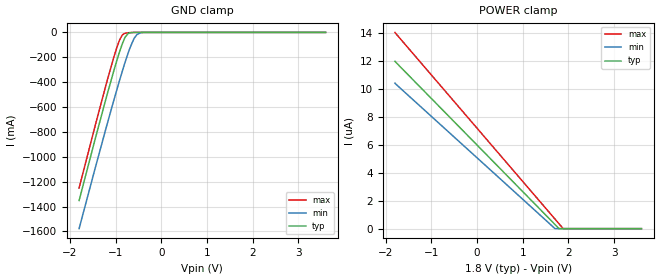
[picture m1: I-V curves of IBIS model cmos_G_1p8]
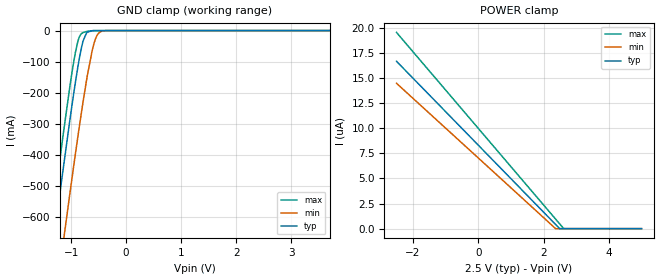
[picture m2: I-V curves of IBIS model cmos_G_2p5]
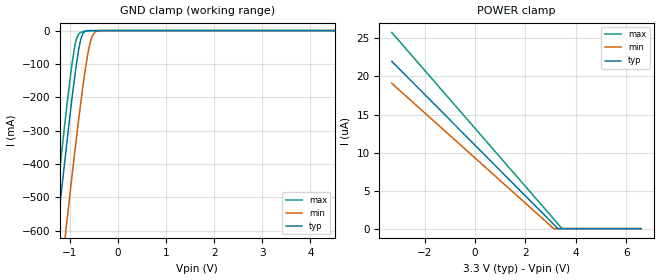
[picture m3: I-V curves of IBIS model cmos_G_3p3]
|Texas Instruments Incorporated
| 1.8V, 2.5V, 3.3V LVCMOS High-Performance Clock Buffer
| Marketing Part # : LMK1C1104
| Voltage Range : 1.71V-3.465V
| Package-type: TSSOP
| #pins/pkg drawing : 8-pin TSSOP
[IBIS Ver] 4.1
[File name] lmk1c1104.ibs
[File Rev] 1.0
[Date] 12/03/2019
[Source]
| Texas Instruments Incorporated.
| 12500 TI Blvd
| Dallas, TX -75243
[Notes] Revision History:
| Rev 1.0: 12/03/2019
| - Initial version of the model
| - Model generated from simulations in SPECTRE
| - C_comp although listed in numerical order of value are
| obtained from varying PVT conditions. For PVT conditions for
| each specific value refer the buffer description under
| respective [Model]. IBIS model user is responsible for using
| appropriate C_comp to simulate for Signal Integrity.
| - Warnings regarding combined Non-monotonicity of various models have been
| reviewed and considered minor and can be ignored.
| - Model names with a trailing _1p8 contain the model for
| 1.8V operation. Model names with a trailing _2p5 contain the model
| for 2.5V operation. Model names with a trailing _3p3 contain the model
| for 3.3V operation.
[Disclaimer]
| This model is designed as an aid for customers of Texas Instruments.
| TI and its licensors and suppliers make no warranties, either expressed
| or implied, with respect to this model, including the warranties of
| merchantability or fitness for a particular purpose. The model is
| provided solely on an "as is" basis. The entire risk as to its quality
| and performance is with the customer.
| This model is subject to change without notice. Texas Instruments
| Incorporated is not responsible for updating this model.
[Copyright]
(C) Copyright 2019 Texas Instruments Incorporated. All rights reserved.
|   Component LMK1C1104
[Component]   LMK1C1104
[Manufacturer]  Texas Instruments Incorporated
[Package] |8-pin TSSOP package
| variable   typ   min   max
R_pkg   30m   24m   36m
L_pkg   2.7n   2.16n   3.24n
C_pkg   0.3p   0.24p   0.36p
|-------------------------PIN------------------------------------------------
[Pin]  signal_name   model_name   R_pin   L_pin   C_pin
1   CLKIN   cmos_in   29.96m   2.73n   0.342p
2   1G   cmos_G   62.4m   2.785n   0.311p
3   Y0   cmos_out   31.6m   2.44n   0.34p
4   GND   GND   30.49m   2.81n   0.34p
5   Y2   cmos_out   29.7m   2.734n   0.34p
6   VDD   POWER   21.634m   2.32n   0.377p
7   Y3   cmos_out   31.9m   2.445n   0.35p
8   Y1   cmos_out   31.16m   2.86n   0.34p
[Model Selector]   cmos_in
cmos_in_1p8   cmos input model at 1.8V
cmos_in_2p5   cmos input model at 2.5V
cmos_in_3p3   cmos input model at 3.3V
[Model Selector]   cmos_G
cmos_G_1p8   cmos 1G model at 1.8V
cmos_G_2p5   cmos 1G model at 2.5V
cmos_G_3p3   cmos 1G model at 3.3V
[Model Selector]   cmos_out
cmos_out_1p8   cmos output model at 1.8V
cmos_out_2p5   cmos output model at 2.5V
cmos_out_3p3   cmos output model at 3.3V
| Models and submodels in the file (9): cmos_G_1p8 (Input), cmos_G_2p5 (Input), cmos_G_3p3 (Input), cmos_in_1p8 (Input), cmos_in_2p5 (Input), cmos_in_3p3 (Input), cmos_out_1p8 (Output), cmos_out_2p5 (Output), cmos_out_3p3 (Output)
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[Model]   cmos_G_1p8
Model_type   Input
Vinl = 0.45
Vinh = 1.35
|   typ   min   max
C_comp   2.69pF   2.601pF   2.886pF
[Voltage Range]   1.8   1.71   1.89
[Temperature Range]   25   150   -40
[Power Clamp Reference]   1.8   1.71   1.89
[GND Clamp Reference]   0   0   0
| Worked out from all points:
|   GND clamp passes 1 mA (typ) near -0.62 V on its own axis
[GND Clamp]
|   Voltage   I(typ)   I(min)   I(max)
-1.8V     -1.351A    -1.577A    -1.251A
-1.211V   -533.8mA   -771.9mA   -423.2mA
-1.039V   -307.6mA   -544.8mA   -198.6mA
-925.2mV  -169.5mA   -400.5mA   -72.4mA
-844.2mV  -83.24mA   -301.1mA   -17.85mA
-784.8mV  -34.97mA   -231.3mA   -6.505mA
-725.4mV  -8.825mA   -165.5mA   -3.073mA
-601.2mV  -280.2uA   -52.64mA   -316uA
-531mV    -45.76uA   -16.45mA   -52.62uA
-444.6mV  -5.415uA   -2.134mA   -5.055uA
-342mV    -1.279uA   -137.3uA   -1.351uA
3.6V      0A         0A         0A
[POWER Clamp]
|   Voltage   I(typ)   I(min)   I(max)
-1.8V     12uA       10.43uA    14.07uA
1.699V    319.7nA    16.08nA    712.2nA
1.791V    13.1nA     0A         361.8nA
1.883V    0A         0A         11.28nA
3.6V      0A         0A         0A
[Model]   cmos_G_2p5
Model_type   Input
Vinl = 0.625
Vinh = 1.875
|   typ   min   max
C_comp   2.623pF   2.472pF   2.811pF
[Voltage Range]   2.5   2.375   2.625
[Temperature Range]   25   150   -40
[Power Clamp Reference]   2.5   2.375   2.625
[GND Clamp Reference]   0   0   0
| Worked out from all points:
|   GND clamp passes 1 mA (typ) near -0.63 V on its own axis
[GND Clamp]
|   Voltage   I(typ)   I(min)   I(max)
-2.5V     -2.35A     -2.56A     -2.262A
-1.48V    -901.5mA   -1.135A    -794.9mA
-1.232V   -562.1mA   -800.1mA   -451.7mA
-1.157V   -462mA     -700.4mA   -351.1mA
-1.022V   -287.3mA   -524mA     -179.1mA
-925mV    -169.3mA   -400.2mA   -72.21mA
-857.5mV  -96.2mA    -317.1mA   -23.38mA
-782.5mV  -33.5mA    -228.7mA   -6.31mA
-707.5mV  -5.337mA   -146.7mA   -2.398mA
-587.5mV  -196.1uA   -43.59mA   -227.3uA
-430mV    -3.965uA   -1.456mA   -3.623uA
5V        0A         0A         0A
[POWER Clamp]
|   Voltage   I(typ)   I(min)   I(max)
-2.5V     16.67uA    14.48uA    19.54uA
2.36V     444.4nA    22.36nA    989.6nA
2.487V    18.24nA    0A         502.7nA
2.615V    0A         0A         15.69nA
5V        0A         0A         0A
[Model]   cmos_G_3p3
Model_type   Input
Vinl = 0.825
Vinh = 2.475
|   typ   min   max
C_comp   2.566pF   2.41pF   2.75pF
[Voltage Range]   3.3   3.135   3.465
[Temperature Range]   25   150   -40
[Power Clamp Reference]   3.3   3.135   3.465
[GND Clamp Reference]   0   0   0
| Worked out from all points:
|   GND clamp passes 1 mA (typ) near -0.65 V on its own axis
[GND Clamp]
|   Voltage   I(typ)   I(min)   I(max)
-3.3V     -3.502A    -3.695A    -3.427A
-1.429V   -830.6mA   -1.065A    -723.1mA
-1.3V     -653.8mA   -891mA     -544.2mA
-1.28V    -626.9mA   -864.3mA   -517mA
-1.211V   -533.4mA   -771.5mA   -422.8mA
-1.102V   -389.4mA   -627.6mA   -278.9mA
-1.033V   -300.4mA   -537.4mA   -191.7mA
-904.2mV  -145.7mA   -374.3mA   -53.93mA
-765.6mV  -23.82mA   -209.5mA   -5.096mA
-587.4mV  -195.6uA   -43.53mA   -226.7uA
-419.1mV  -3.199uA   -1.092mA   -2.912uA
6.6V      0A         0A         0A
[POWER Clamp]
|   Voltage   I(typ)   I(min)   I(max)
-3.3V     22uA       19.11uA    25.8uA
3.115V    587nA      29.49nA    1.307uA
3.284V    24.16nA    0A         663.9nA
3.452V    0A         0A         20.76nA
6.6V      0A         0A         0A
